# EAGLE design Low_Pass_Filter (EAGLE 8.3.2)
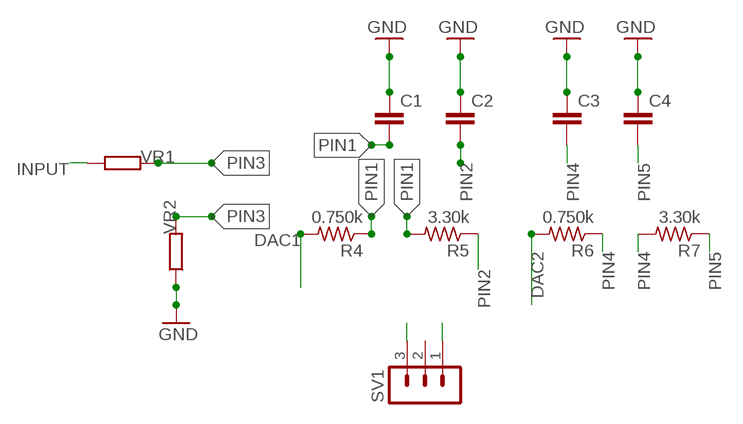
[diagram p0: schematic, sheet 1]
R2 (R): VR2: 3.3K
R3 (R): VR1: 5K

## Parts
C1  C27/9  [C27.5B9]
C2  C27/9  [C27.5B9]
C3  C27/9  [C27.5B9]
C4  C27/9  [C27.5B9]
R4  0.750k  R-US_0309/10  [0309/10]
R5  3.30k  R-US_0309/10  [0309/10]
R6  0.750k  R-US_0309/10  [0309/10]
R7  3.30k  R-US_0309/10  [0309/10]
SV1  MA03-1  [MA03-1]

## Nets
DAC1: R4.2 SV1.3
DAC2: R6.2 SV1.1
GND: C1.1
GND1: C2.1
GND2: C3.1
GND3: C4.1
PIN1: C1.2 R4.1 R5.2
PIN2: C2.2 R5.1
PIN4: C3.2 R6.1 R7.2
PIN5: C4.2 R7.1
Unconnected: SV1.2

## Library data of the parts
C1-C4 = capacitor-wima:C: CAPACITOR
R4-R7 = resistor:R-US_: RESISTOR, American symbol
SV1 = con-lstb:MA03-1: PIN HEADER; OC_FARNELL: unknown; OC_NEWARK: unknown

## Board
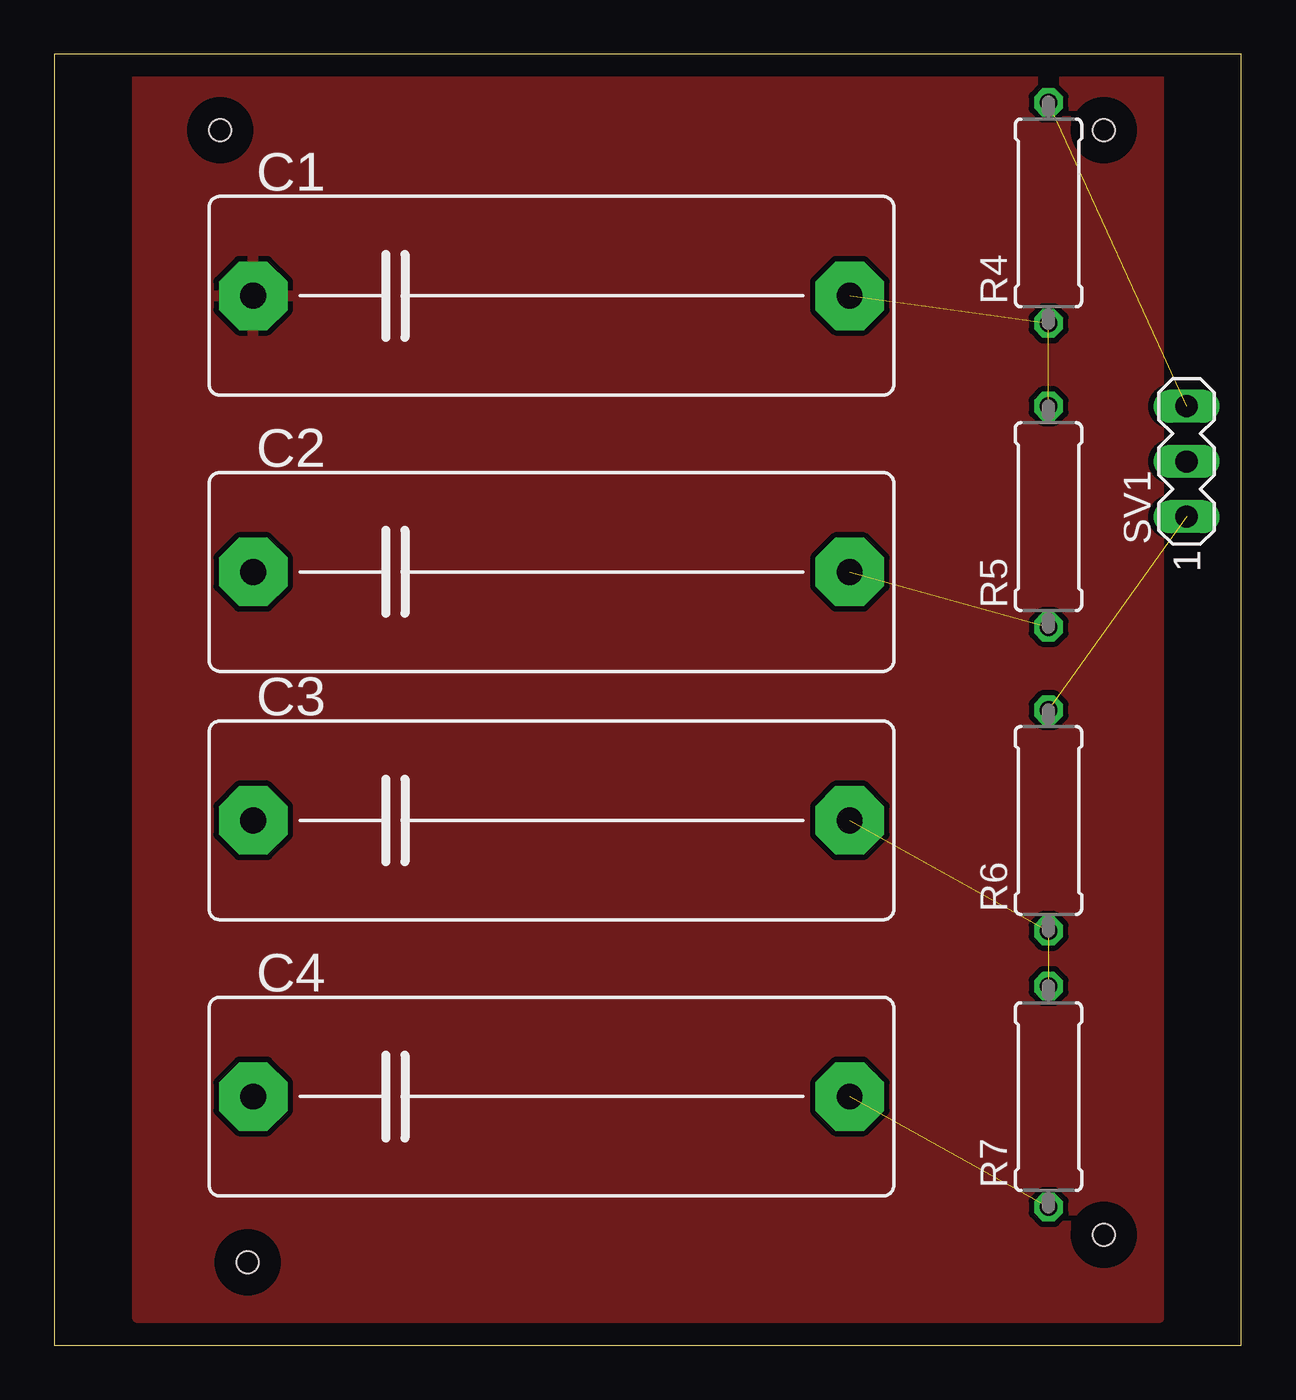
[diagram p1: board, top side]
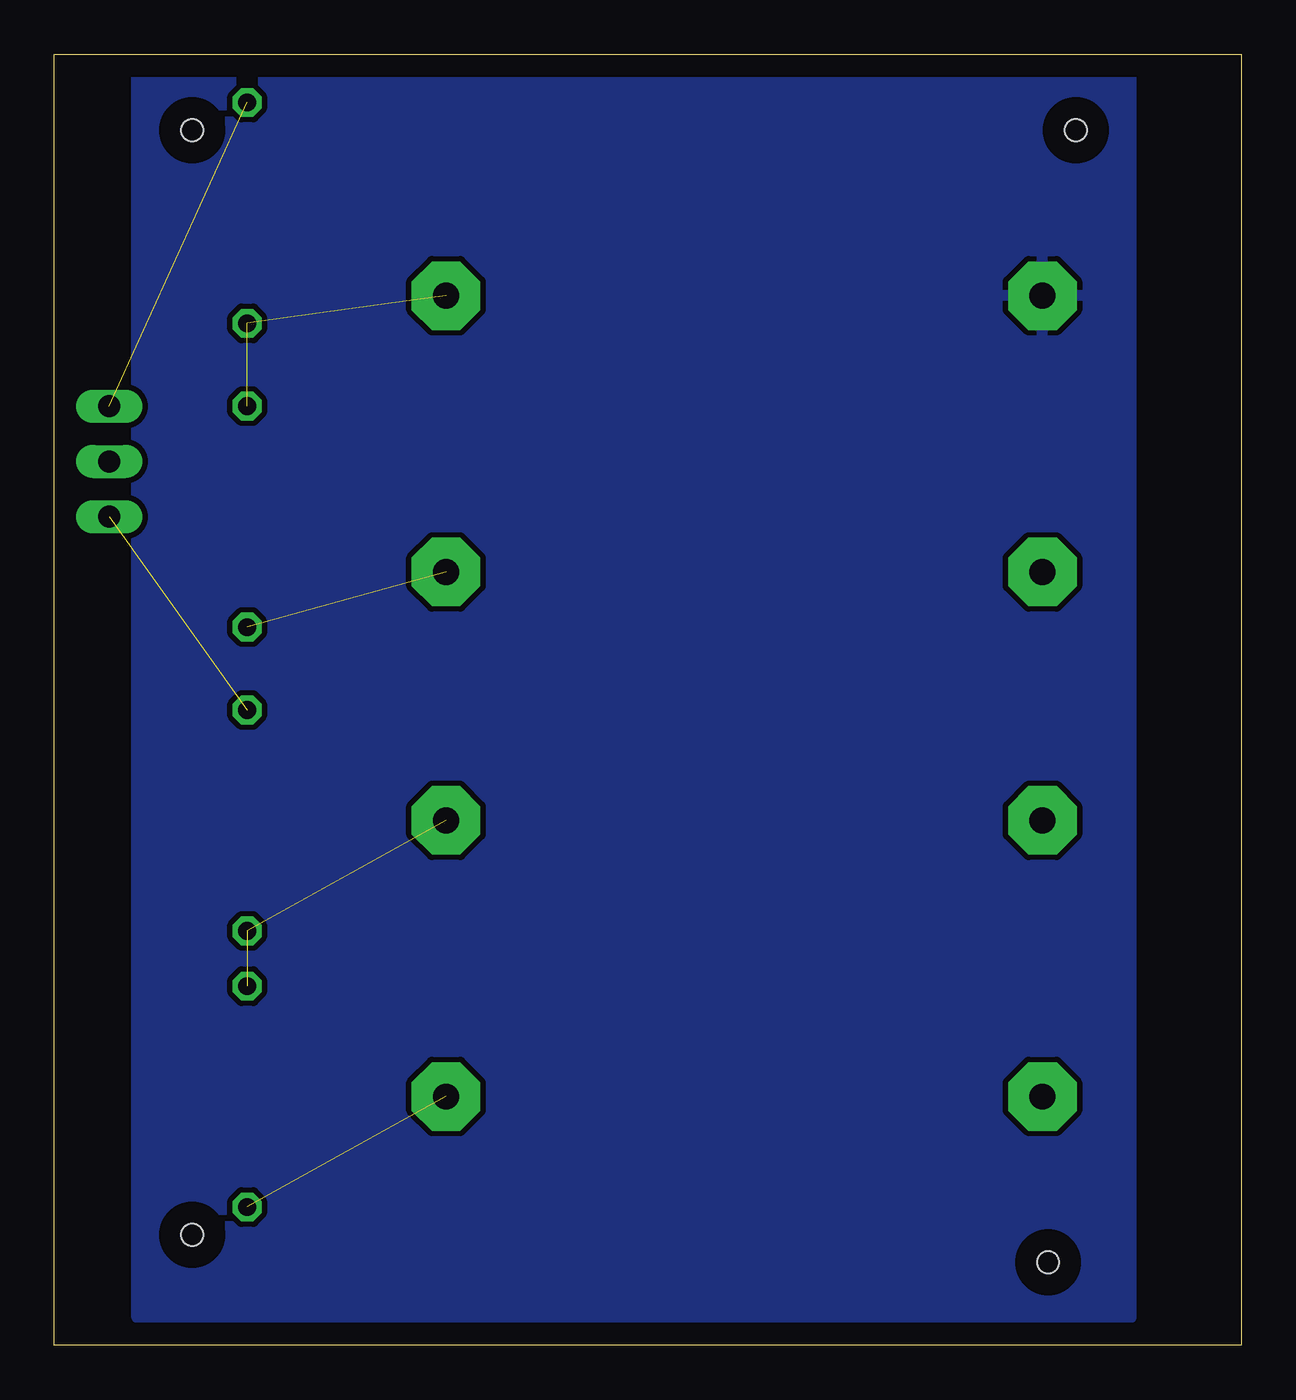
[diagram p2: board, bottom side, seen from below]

Size 54.59 x 59.36 mm. Coordinates in mm from the lower left corner, seen from the top.
Outline: 0,0 54.59,0 54.59,59.36 0,59.36 0,0
Copper layers (1*16): Top 0.035mm / dielectric 1.5mm / Bottom 0.035mm
Design rules "default *": minimum track width 6mil, minimum drill 0.35mm, track to track 10mil, track to pad 10mil, pad to pad 10mil, via to via 10mil, smd to smd 10mil, copper to edge 40mil, drill to drill 6mil, minimum pad ring 10mil, minimum via ring 8mil, stop-mask expansion 4mil, vias tented up to drill 0mil, thermal gap 10mil
Holes 1 mm at 7.62,55.88 8.89,3.81 48.26,5.08 48.26,55.88

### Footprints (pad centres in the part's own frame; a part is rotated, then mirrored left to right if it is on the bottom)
C27.5B9 = drill 1.194 pad 3.15 octagon: 1 -13.716,0; 2 13.716,0
0309/10 = drill 0.813 octagon: 1 -5.08,0; 2 5.08,0
MA03-1 = drill 1.016 long: 1 -2.54,0; 2 0,0; 3 2.54,0

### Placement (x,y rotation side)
C1  22.86,48.26 0 top
C2  22.86,35.56 0 top
C3  22.86,24.13 0 top
C4  22.86,11.43 0 top
R4  45.72,52.07 90 top
R5  45.72,38.1 90 top
R6  45.72,24.13 90 top
R7  45.72,11.43 90 top
SV1  52.07,40.64 90 top

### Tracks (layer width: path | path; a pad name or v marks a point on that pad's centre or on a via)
DAC1  (1 unrouted)
DAC2  (1 unrouted)
GND
  pour Bottom: 5.08,58.42 5.08,1.27 50.8,1.27 50.8,58.42
  pour Top: 3.81,58.42 3.81,1.27 50.8,1.27 50.8,58.42
PIN1  (2 unrouted)
PIN2  (1 unrouted)
PIN4  (2 unrouted)
PIN5  (1 unrouted)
